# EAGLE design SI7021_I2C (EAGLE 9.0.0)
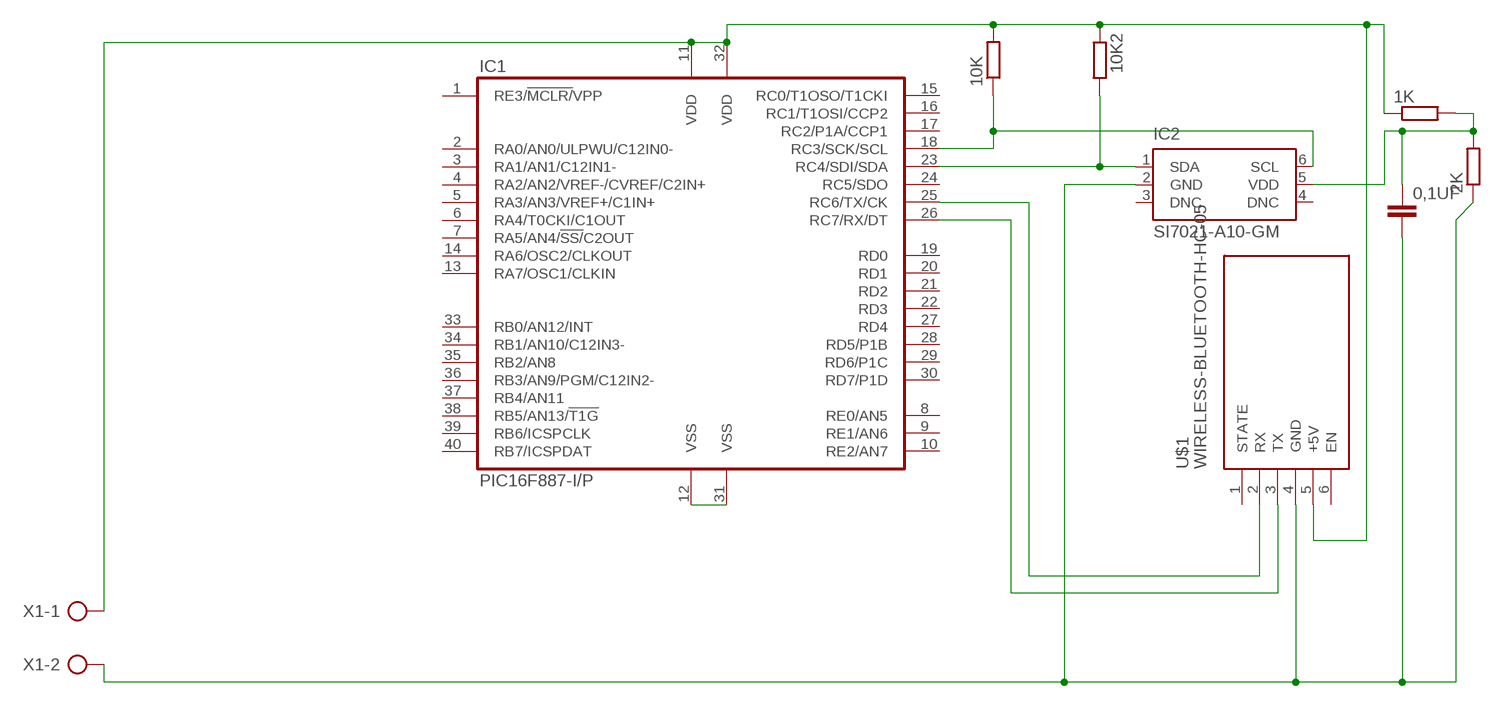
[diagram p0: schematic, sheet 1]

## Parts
0,1UF  C-EU050-030X075  [C050-030X075]
1K  R-EU_0207/12  [0207/12]
2K  R-EU_0207/12  [0207/12]
10K  R-EU_0207/12  [0207/12]
10K2  R-EU_0207/12  [0207/12]
IC1  PIC16F887-I/P  [DIL40]
IC2  SI7021-A10-GM  [DFN6-3X3]
U$1  WIRELESS-BLUETOOTH-HC-05  [WIRELESS-BLUETOOTH-HC-05]
X1  AK500/2  [AK500/2]

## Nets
N$1: IC1.25(RC6/TX/CK) U$1.2(RX)
N$2: IC1.12(VSS) IC1.31(VSS)
N$3: 0,1UF.1 1K.2 2K.2 IC2.5(VDD)
N$4: 0,1UF.2 2K.1 IC2.2(GND) U$1.4(GND) X1.2
N$5: 1K.1 10K2.1 10K.2 IC1.11(VDD) IC1.32(VDD) U$1.5(+5V) X1.1
N$6: IC1.26(RC7/RX/DT) U$1.3(TX)
N$7: 10K2.2 IC1.23(RC4/SDI/SDA) IC2.1(SDA)
N$8: 10K.1 IC1.18(RC3/SCK/SCL) IC2.6(SCL)
Unconnected: IC1.1(RE3/!MCLR/!VPP) IC1.2(RA0/AN0/ULPWU/C12IN0-) IC1.3(RA1/AN1/C12IN1-) IC1.4(RA2/AN2/VREF-/CVREF/C2IN+) IC1.5(RA3/AN3/VREF+/C1IN+) IC1.6(RA4/T0CKI/C1OUT) IC1.7(RA5/AN4/!SS/!C2OUT) IC1.8(RE0/AN5) IC1.9(RE1/AN6) IC1.10(RE2/AN7) IC1.13(RA7/OSC1/CLKIN) IC1.14(RA6/OSC2/CLKOUT) IC1.15(RC0/T1OSO/T1CKI) IC1.16(RC1/T1OSI/CCP2) IC1.17(RC2/P1A/CCP1) IC1.19(RD0) IC1.20(RD1) IC1.21(RD2) IC1.22(RD3) IC1.24(RC5/SDO) IC1.27(RD4) IC1.28(RD5/P1B) IC1.29(RD6/P1C) IC1.30(RD7/P1D) IC1.33(RB0/AN12/INT) IC1.34(RB1/AN10/C12IN3-) IC1.35(RB2/AN8) IC1.36(RB3/AN9/PGM/C12IN2-) IC1.37(RB4/AN11) IC1.38(RB5/AN13/!T1G) IC1.39(RB6/ICSPCLK) IC1.40(RB7/ICSPDAT) IC2.3(DNC) IC2.4(DNC) U$1.1(STATE) U$1.6(EN)

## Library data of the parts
0,1UF = rcl:C-EU: CAPACITOR, European symbol; SPICEPREFIX: C
1K 2K 10K 10K2 = rcl:R-EU_: RESISTOR, European symbol; SPICEPREFIX: R
IC1 = microchip-pic16f887:PIC16F887: The library has been designed by Richard Magdycz
IC2 = si70xx-10:SI7021-*: I2C Humidity and Temperature Sensor Source: http://www.silabs.com/Support%20Documents/TechnicalDocs/Si7021.pdf; MF: Silicon Labs; MPN: Si7021-A10-GM; OC_FARNELL: 2422571; OC_NEWARK: 55X3111
U$1 = diy-modules:WIRELESS-BLUETOOTH-HC-05: Bluetooth Transceiver Module based on HC-05 board Tutorial is available here: https://arduino-info.wikispaces.com/BlueTooth-HC05-HC06-Modules-How-To Click here to find device on ebay.com
X1 = con-ptr500:AK500/2: CONNECTOR; OC_FARNELL: unknown; OC_NEWARK: unknown

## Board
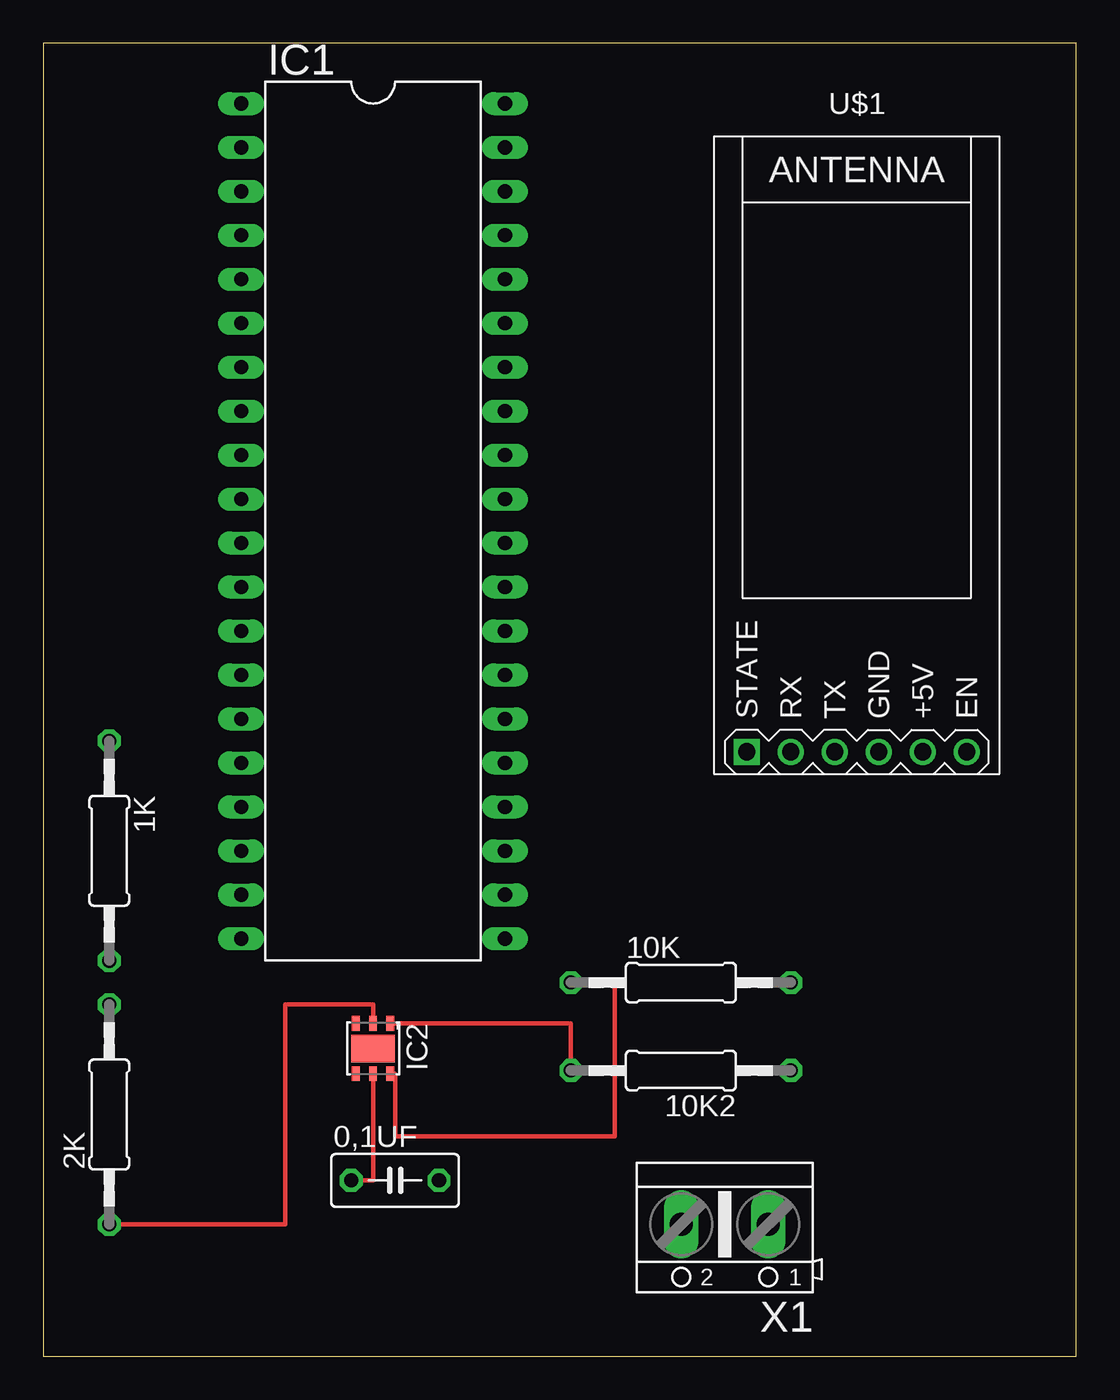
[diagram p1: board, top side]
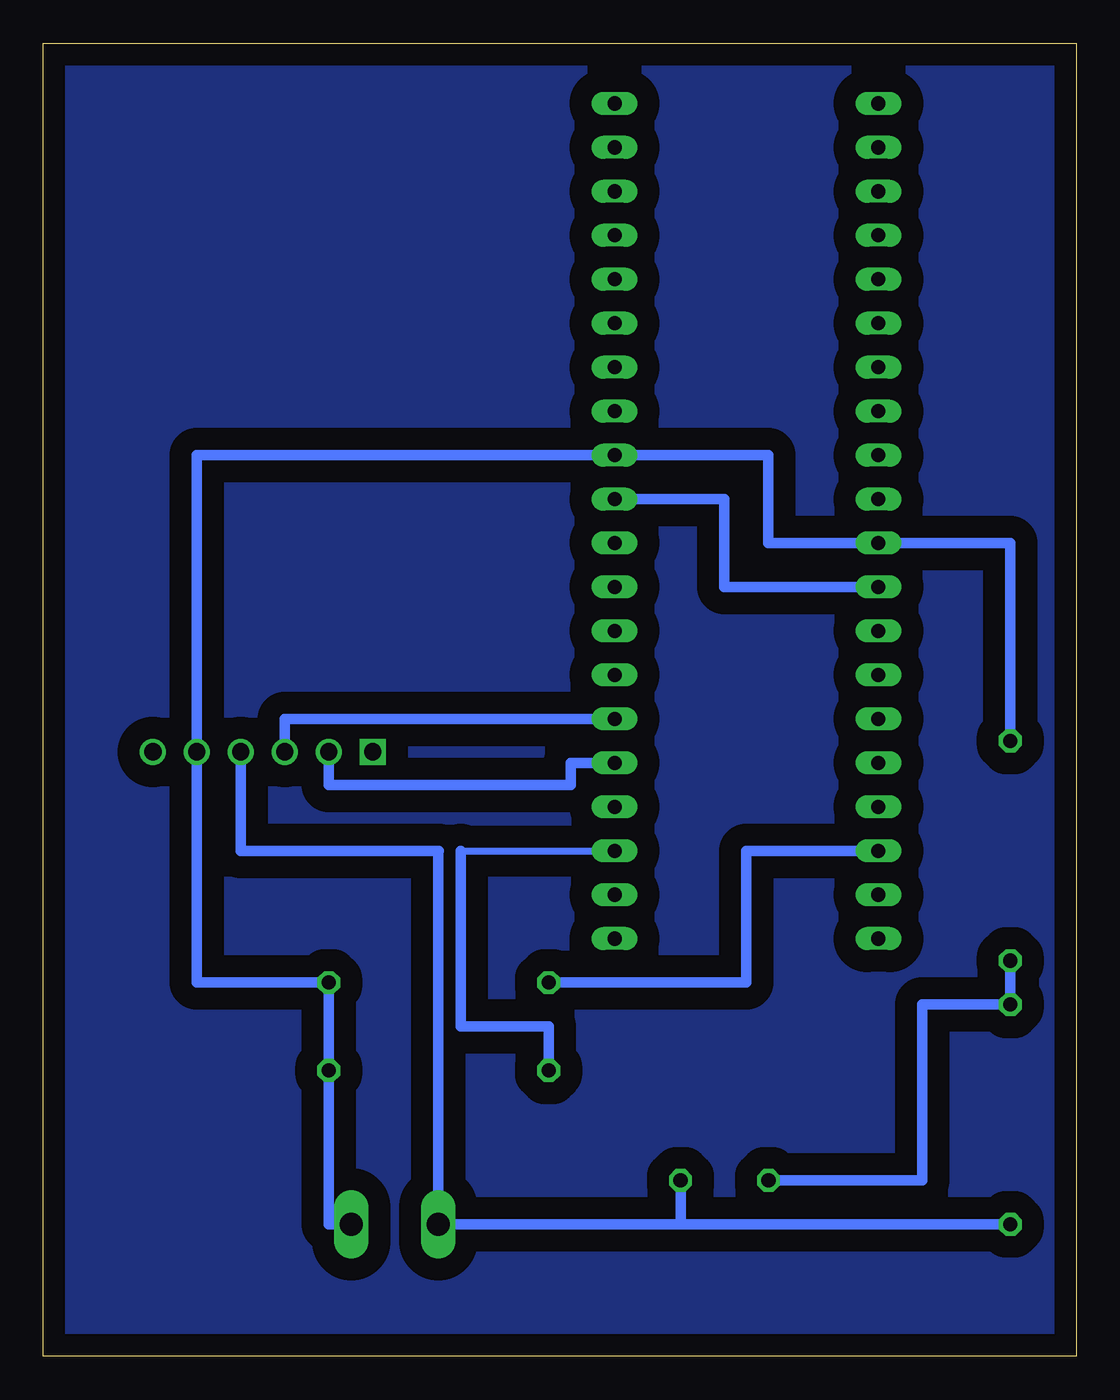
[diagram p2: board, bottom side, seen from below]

Size 59.67 x 75.87 mm. Coordinates in mm from the lower left corner, seen from the top.
Outline: 0,0 59.67,0 59.67,75.87 0,75.87 0,0
Copper layers (1*16): Top 0.035mm / dielectric 1.5mm / Bottom 0.035mm
Design rules "default": minimum track width 6mil, minimum drill 0.35mm, track to track 6mil, track to pad 6mil, pad to pad 6mil, via to via 6mil, smd to smd 6mil, copper to edge 40mil, drill to drill 6mil, minimum pad ring 10mil, minimum via ring 8mil, stop-mask expansion 4mil, vias tented up to drill 0mil, thermal gap 10mil

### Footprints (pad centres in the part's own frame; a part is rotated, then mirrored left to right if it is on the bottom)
C050-030X075 = drill 0.813 octagon: 1 -2.54,0; 2 2.54,0
0207/12 = drill 0.813 octagon: 1 -6.35,0; 2 6.35,0
DIL40 = drill 0.813 long: 1 -24.13,-7.62; 2 -21.59,-7.62; 3 -19.05,-7.62; 4 -16.51,-7.62; 5 -13.97,-7.62; 6 -11.43,-7.62; 7 -8.89,-7.62; 8 -6.35,-7.62; 9 -3.81,-7.62; 10 -1.27,-7.62; 11 1.27,-7.62; 12 3.81,-7.62; 13 6.35,-7.62; 14 8.89,-7.62; 15 11.43,-7.62; 16 13.97,-7.62; 17 16.51,-7.62; 18 19.05,-7.62; 19 21.59,-7.62; 20 24.13,-7.62; 21 24.13,7.62; 22 21.59,7.62; 23 19.05,7.62; 24 16.51,7.62; 25 13.97,7.62; 26 11.43,7.62; 27 8.89,7.62; 28 6.35,7.62; 29 3.81,7.62; 30 1.27,7.62; 31 -1.27,7.62; 32 -3.81,7.62; 33 -6.35,7.62; 34 -8.89,7.62; 35 -11.43,7.62; 36 -13.97,7.62; 37 -16.51,7.62; 38 -19.05,7.62; 39 -21.59,7.62; 40 -24.13,7.62
DFN6-3X3 = smd 0.85 x 0.45: 1 -1.45,1; 2 -1.45,0; 3 -1.45,-1; 4 1.45,-1; 5 1.45,0; 6 1.45,1 | smd 1.6 x 2.5: EXP 0,0
WIRELESS-BLUETOOTH-HC-05 = drill 1 square: 1 -6.35,-17.145 | drill 1: 2 -3.81,-17.145; 3 -1.27,-17.145; 4 1.27,-17.145; 5 3.81,-17.145; 6 6.35,-17.145
AK500/2 = drill 1.321 long: 1 -2.515,0; 2 2.515,0

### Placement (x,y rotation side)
0,1UF  20.32,10.16 0 top
1K  3.81,29.21 270 top
2K  3.81,13.97 90 top
10K  36.83,21.59 0 top
10K2  36.83,16.51 180 top
IC1  19.05,48.26 270 top
IC2  19.05,17.78 270 top
U$1  46.99,52.07 0 top
X1  39.37,7.62 180 top

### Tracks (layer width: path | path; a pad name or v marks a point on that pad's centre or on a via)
N$1
  Bottom 0.61: U$1.2 43.18,33.02 29.21,33.02 29.21,34.29 IC1.25
N$2
  Bottom 0.61: IC1.31 20.32,49.53 20.32,44.45 IC1.12
N$3
  Top 0.254: IC2.5 19.05,10.16 0,1UF.1
  Bottom 0.61: 1K.2 2K.2 8.89,20.32 8.89,10.16 0,1UF.1
N$4
  Top 0.254: IC2.2 19.05,20.32 13.97,20.32 13.97,7.62 2K.1
  Bottom 0.61: 2K.1 22.86,7.62 | 22.86,7.62 0,1UF.2 | 22.86,7.62 X1.2 36.86,29.21 | 36.86,29.21 36.83,29.21 | 36.86,29.21 48.26,29.21 U$1.4
N$5
  Bottom 0.61: 1K.1 3.81,46.99 IC1.11 17.78,46.99 17.78,52.07 IC1.32 50.8,52.07 U$1.5 50.8,21.59 10K.2 10K2.1 43.18,7.62 X1.1
N$6
  Bottom 0.61: U$1.3 45.72,36.83 IC1.26
N$7
  Top 0.254: IC2.1 30.48,19.23 10K2.2
  Bottom 0.406: 35.56,29.21 IC1.23
  Bottom 0.61: 10K2.2 30.48,19.05 35.56,19.05 35.56,29.21
N$8
  Top 0.254: IC2.6 20.32,16.33 20.32,12.7 33.02,12.7 33.02,21.59 10K.1
  Bottom 0.61: 10K.1 19.05,21.59 19.05,29.21 IC1.18
N$9
  pour Bottom (isolate 1.27): 0,76.2 59.69,76.2 59.69,0 0,0

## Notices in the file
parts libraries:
si70xx-10: (c) 2014 Samuel Lourenço
diy-modules: Released under the Creative Commons Attribution 4.0 International License: http://creativecommons.org/licenses/by/4.0
